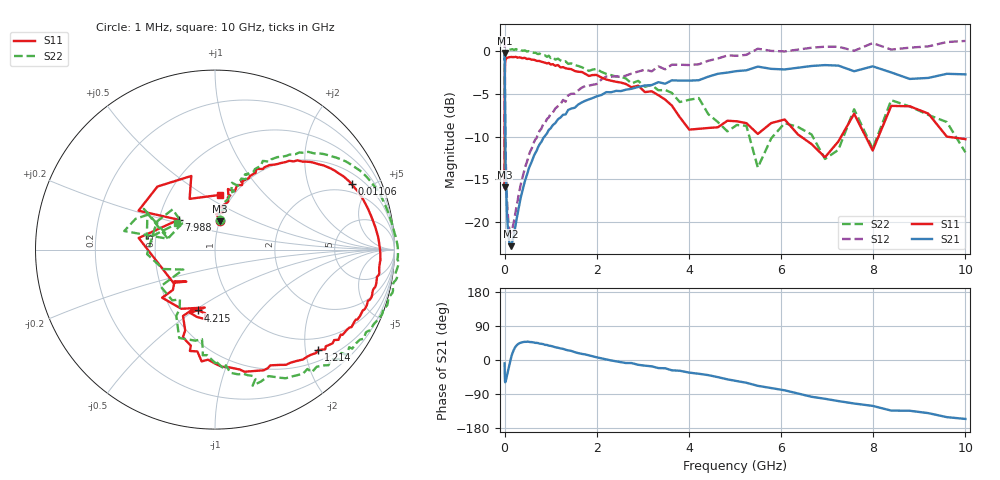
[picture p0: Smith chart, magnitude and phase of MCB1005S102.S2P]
!Agilent Technologies,E5071C,MY46111244,A.11.31
!Date: Tue May 07 15:03:32 2019
!Data & Calibration Information:
!Freq	S11:SOLT2(ON)	S21:SOLT2(ON)	S12:SOLT2(ON)	S22:SOLT2(ON)
# Hz S dB R 50
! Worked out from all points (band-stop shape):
!   201 points, 1 MHz to 10 GHz, reference 50 ohm
!   highest |S21| = -0.23 dB at 1.212 MHz (marker M1); lowest = -22.8 dB at 132.5 MHz (marker M2)
!   |S21| within 3 dB of the highest: 4.304 GHz to 8.777 GHz (4.472 GHz wide, 68.4 % of centre); 8.897 GHz to end of sweep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
!   lowest |S11| = -15.9 dB at 1 MHz (marker M3), VSWR 1.38, Z = 50.3 + j16.2 ohm
!   |S11| at or under -10 dB: start of sweep to 2.012 MHz; 6.433 GHz to 7.303 GHz (870.7 MHz wide, 12.7 % of centre); 9.597 GHz to end of sweep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
!   |S22| runs from -15.6 to 0.2 dB; largest |S21 - S12| = 0.52
!   S11 on the Smith chart (normalised r, x): 1 MHz: 1.01, +0.32; 11.06 MHz: 1.52, +3.85; 1.214 GHz: 0.72, -2.26; 4.215 GHz: 0.67, -0.52; 7.988 GHz: 0.63, +0.23; 10 GHz: 0.87, +0.59
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1000000  -15.93 79.9  -0.40 -8.7  1.05 -9.6  -15.61 80.5
1212171  -14.14 87.8  -0.23 -11.2  1.23 -12.1  -13.47 83.6
4810209  -4.04 51.0  -2.52 -38.7  -1.01 -39.6  -3.15 49.8
1.106086e7  -1.47 25.5  -7.53 -57.3  -5.98 -58.0  -0.52 24.7
2.206931e7  -1.02 12.3  -12.87 -57.0  -11.33 -57.4  -0.11 11.5
1.047129e8  -0.72 -0.9  -22.36 -13.4  -20.84 -13.4  0.17 -1.7
1.324842e8  -0.70 -2.9  -22.79 1.5  -21.28 1.6  0.16 -3.2
4.810209e8  -0.93 -18.4  -14.60 48.0  -13.04 49.1  -0.05 -19.4
1.213756e9  -1.92 -44.3  -7.77 30.6  -6.22 33.0  -1.10 -47.1
2.206931e9  -3.33 -78.4  -4.80 1.3  -2.98 7.2  -2.67 -73.2
3.484689e9  -5.67 -110.1  -3.82 -21.8  -2.14 -12.8  -4.55 -96.6
4.215088e9  -9.08 -105.2  -3.41 -36.3  -1.55 -25.4  -5.49 -112.1
5.248075e9  -8.42 -111.5  -2.25 -60.1  -0.45 -47.1  -8.74 -145.9
5.495409e9  -9.68 -100.0  -1.82 -68.1  0.27 -55.2  -13.61 -147.8
6.078392e9  -8.00 -137.7  -2.15 -80.0  -0.05 -65.5  -8.42 -176.2
6.661376e9  -10.87 -142.0  -1.75 -97.0  0.38 -80.6  -9.74 136.6
6.952868e9  -12.41 -131.9  -1.64 -102.3  0.50 -84.8  -12.61 141.0
7.585776e9  -7.33 171.4  -2.36 -114.8  0.03 -99.1  -6.80 150.2
7.988146e9  -11.62 140.6  -1.79 -121.1  0.93 -103.7  -11.41 167.1
8.390517e9  -6.41 153.0  -2.50 -133.5  0.17 -114.6  -5.74 168.5
9.195259e9  -7.31 107.9  -3.14 -140.2  0.54 -122.3  -7.46 152.8
1e10  -10.29 85.0  -2.73 -155.6  1.17 -135.8  -11.83 145.4
